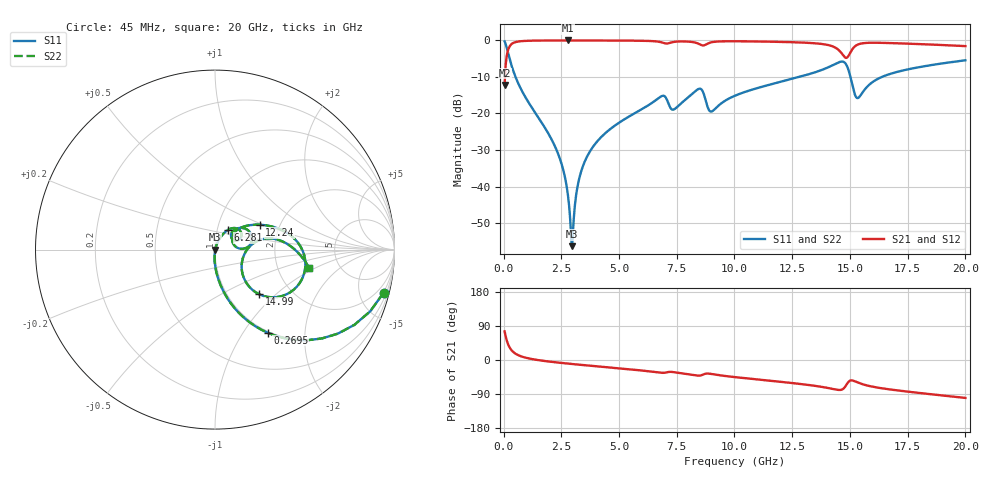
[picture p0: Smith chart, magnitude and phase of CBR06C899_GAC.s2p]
! S-parameter model data by Modelithics Inc.  support@modelithics.com 813-866-6335  Tampa FL USA
! S-Parameter data specifications:
! Substrate: 20-mil Rogers 4350B, substrate thickness, H=0.508mm, Dielectric constant, Er=3.75
! PCB Mounting Pad Footprint: Pad width, PadW=0.85mm , Pad length, PadL=0.64mm , Pad gap, PadG (edge-to-edge)=0.62mm , Reference planes=1.9mm apart
#  GHz  S  MA  R 50
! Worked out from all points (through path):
!   801 points, 45 MHz to 20 GHz, reference 50 ohm
!   highest |S21| = -0.01 dB at 2.789 GHz (marker M1); lowest = -12.2 dB at 45 MHz (marker M2)
!   group delay of S21, straight-line fit = 14.9 ps
!   lowest |S11| = -56.3 dB at 2.963 GHz (marker M3), VSWR 1.00, Z = 50.2 - j0.0157 ohm
!   |S11| at or under -10 dB: 517.9 MHz to 12.8 GHz (12.28 GHz wide, 184 % of centre); 15.02 GHz to 16.38 GHz (1.362 GHz wide, 8.67 % of centre)
!   |S22| runs from -56.3 to -0.3 dB; largest |S21 - S12| = 0
!   S11 on the Smith chart (normalised r, x): 45 MHz: 0.98, -7.82; 269.5 MHz: 0.98, -1.30; 6.281 GHz: 1.12, +0.25; 12.24 GHz: 1.57, +0.47; 14.99 GHz: 1.39, -0.79; 20 GHz: 3.02, -0.86
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0.045  0.9695 -14.3  0.2451 75.6  0.2451 75.6  0.9695 -14.3
0.269494  0.5479 -57.7  0.836 32.3  0.836 32.3  0.5479 -57.7
0.718481  0.2274 -79.2  0.973 10.6  0.973 10.6  0.2274 -79.2
2.289938  0.03191 -93.9  0.998 -6.3  0.998 -6.3  0.03191 -93.9
2.589262  0.01667 -93.4  0.9983 -8.3  0.9983 -8.3  0.01667 -93.4
2.788813  0.007571 -88.3  0.9983 -9.5  0.9983 -9.5  0.007571 -88.3
2.963419  0.001528 -5.9  0.9983 -10.6  0.9983 -10.6  0.001528 -5.9
3.387462  0.01716 71.5  0.998 -13.0  0.998 -13.0  0.01716 71.5
4.285437  0.04955 69.7  0.9966 -18.1  0.9966 -18.1  0.04955 69.7
6.280938  0.1302 56.9  0.9834 -29.7  0.9834 -29.7  0.1302 56.9
6.704981  0.1617 48.1  0.9614 -32.9  0.9614 -32.9  0.1617 48.1
7.378463  0.1137 37.1  0.9536 -32.1  0.9536 -32.1  0.1137 37.1
8.500931  0.2186 22.1  0.8821 -41.2  0.8821 -41.2  0.2186 22.1
8.999806  0.1063 23.0  0.9421 -36.9  0.9421 -36.9  0.1063 23.0
10.0225  0.1751 41.2  0.9731 -45.2  0.9731 -45.2  0.1751 41.2
12.24249  0.2841 29.2  0.9498 -59.1  0.9498 -59.1  0.2841 29.2
13.36496  0.3558 20.4  0.9188 -67.2  0.9188 -67.2  0.3558 20.4
14.58721  0.5106 -9.5  0.6982 -79.0  0.6982 -79.0  0.5106 -9.5
14.98631  0.3487 -45.4  0.6538 -55.1  0.6538 -55.1  0.3487 -45.4
15.33552  0.1625 -15.5  0.8755 -59.3  0.8755 -59.3  0.1625 -15.5
16.68248  0.3432 9.8  0.9208 -77.3  0.9208 -77.3  0.3432 9.8
20  0.5343 -11.0  0.8356 -100.1  0.8356 -100.1  0.5343 -11.0
